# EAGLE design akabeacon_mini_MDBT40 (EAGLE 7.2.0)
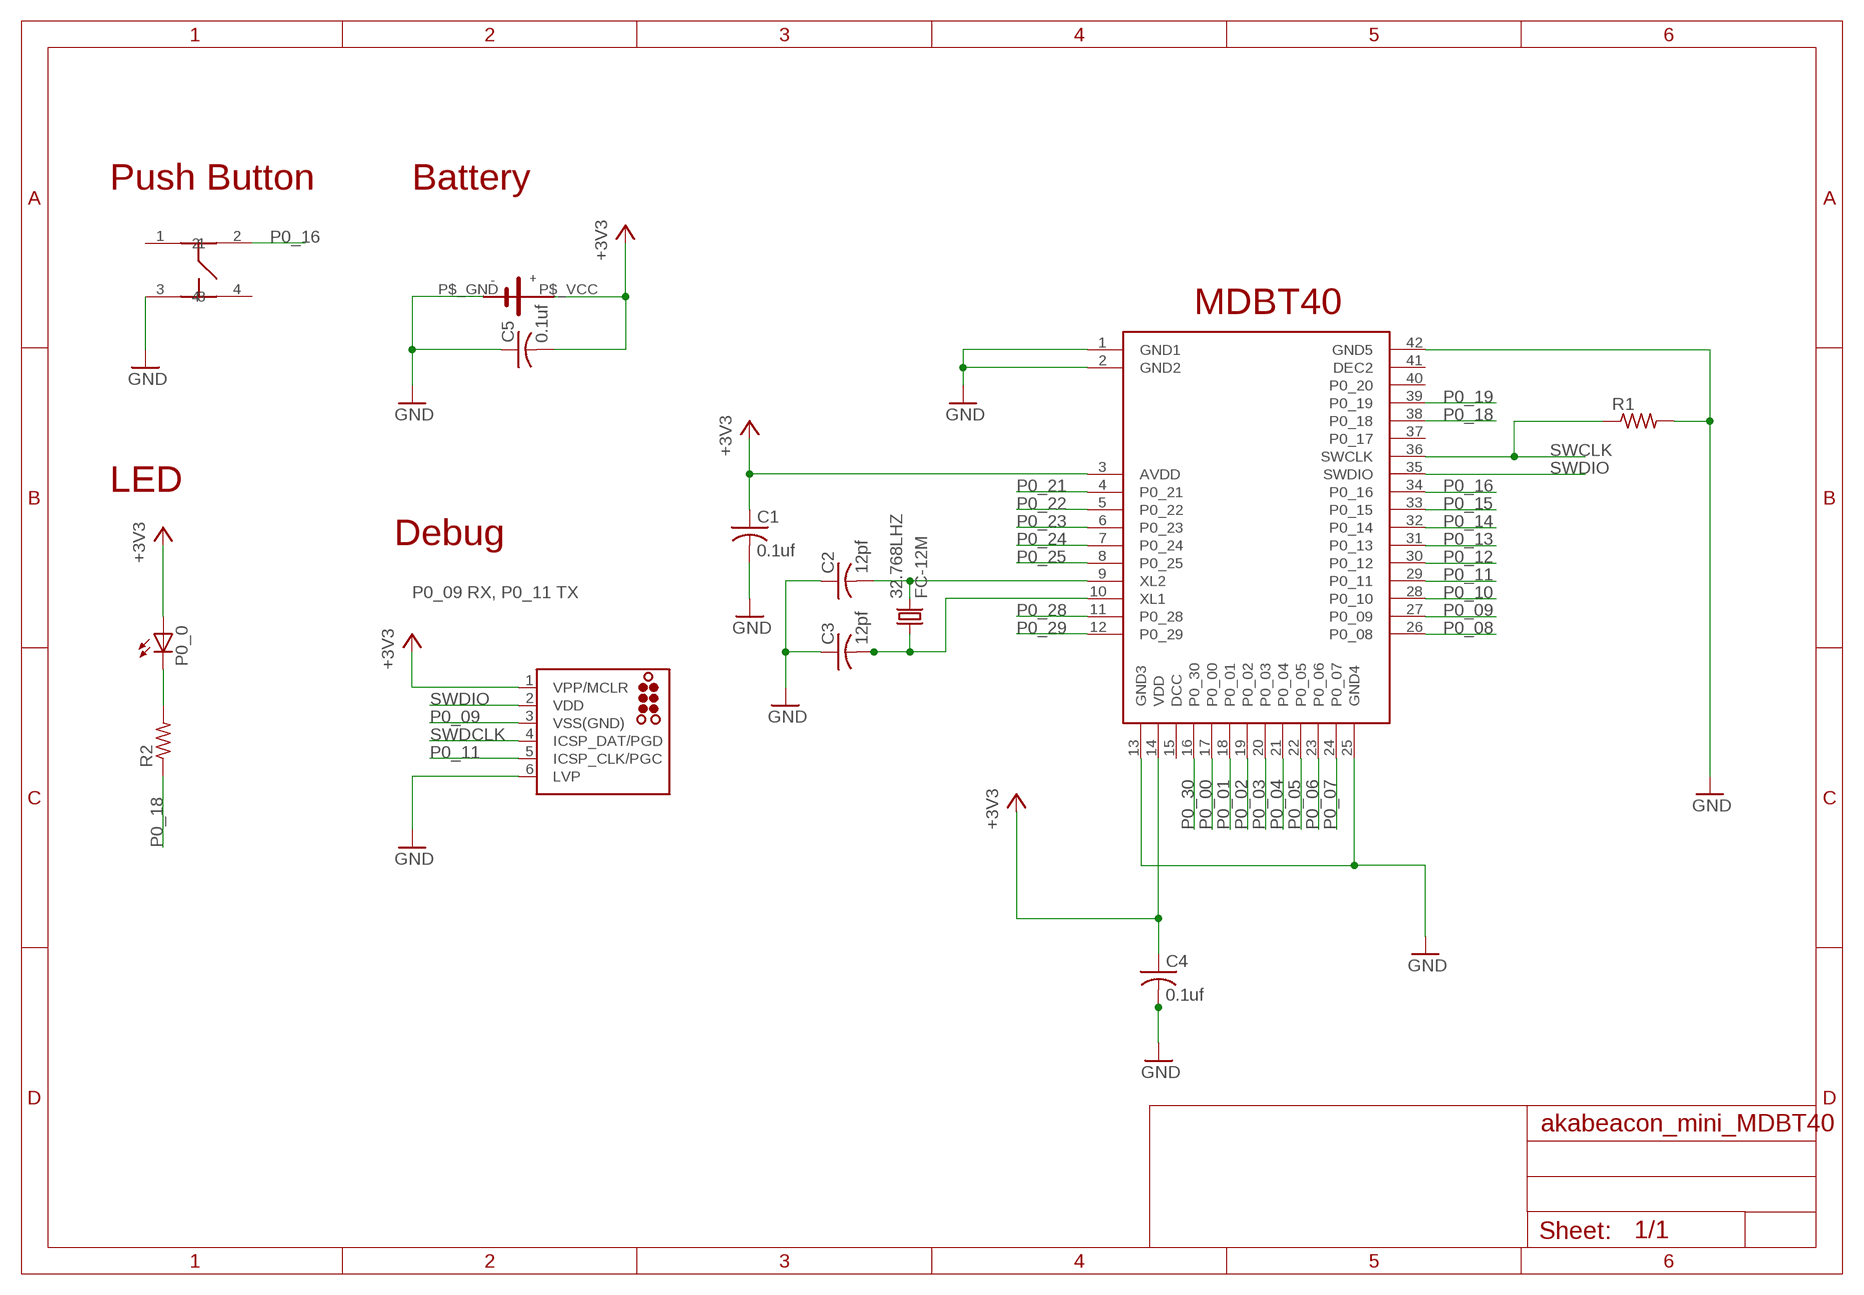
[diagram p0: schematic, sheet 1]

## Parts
32.768LHZ  FC-12M  [FC-12M]
C1  0.1uf  C-USC0603  [C0603]
C2  12pf  C-USC0603  [C0603]
C3  12pf  C-USC0603  [C0603]
C4  0.1uf  C-USC0603  [C0603]
C5  0.1uf  C-USC0603  [C0603]
J2  TC2030-MCP  [TC2030-MCP]
P0_0  LEDCHIP-LED0603  [CHIP-LED0603]
R1  R-US_R0603  [R0603]
R2  R-US_R0603  [R0603]
U$1  RAYTAC-MDBT40  [RAYTAC-MDBT40]
U$3  SMTU2450-BOTTOM-MINI  [SMTU2450-BOTTOM-MINI]
U$5  SWICTH-4P(KMR2)  [SWITCH-4P(KMR2)]

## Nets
+3V3: C1.1 C4.1 C5.2 J2.1(VPP/MCLR) P0_0.A U$1.3(AVDD) U$1.14(VDD) U$3.P$_VCC
GND: C1.2 C2.1 C3.1 C4.2 C5.1 J2.6(LVP) R1.2 U$1.1(GND1) U$1.2(GND2) U$1.13(GND3) U$1.25(GND4) U$1.42(GND5) U$3.P$_GND U$5.3
LED1: P0_0.C R2.2
N$7: 32.768LHZ.2 C2.2 U$1.9(XL2)
N$8: 32.768LHZ.1 C3.2 U$1.10(XL1)
P0_00: U$1.17(P0_00)
P0_01: U$1.18(P0_01)
P0_02: U$1.19(P0_02)
P0_03: U$1.20(P0_03)
P0_04: U$1.21(P0_04)
P0_05: U$1.22(P0_05)
P0_06: U$1.23(P0_06)
P0_07: U$1.24(P0_07)
P0_08: U$1.26(P0_08)
P0_09: J2.3(VSS(GND)) U$1.27(P0_09)
P0_10: U$1.28(P0_10)
P0_11: J2.5(ICSP_CLK/PGC) U$1.29(P0_11)
P0_12: U$1.30(P0_12)
P0_13: U$1.31(P0_13)
P0_14: U$1.32(P0_14)
P0_15: U$1.33(P0_15)
P0_16: U$1.34(P0_16) U$5.2
P0_18: R2.1 U$1.38(P0_18)
P0_19: U$1.39(P0_19)
P0_21: U$1.4(P0_21)
P0_22: U$1.5(P0_22)
P0_23: U$1.6(P0_23)
P0_24: U$1.7(P0_24)
P0_25: U$1.8(P0_25)
P0_28: U$1.11(P0_28)
P0_29: U$1.12(P0_29)
P0_30: U$1.16(P0_30)
SWCLK: R1.1 U$1.36(SWCLK)
SWDCLK: J2.4(ICSP_DAT/PGD)
SWDIO: J2.2(VDD) U$1.35(SWDIO)
Unconnected: U$1.15(DCC) U$1.37(P0_17) U$1.40(P0_20) U$1.41(DEC2) U$5.1 U$5.4

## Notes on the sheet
- Push Button | Battery
- MDBT40
- LED
- Debug
- P0_09 RX, P0_11 TX

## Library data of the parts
32.768LHZ = crystal:FC-12M: kHz RANGE CRYSTAL UNIT
C1-C5 = adafruit:C-US: CAPACITOR, American symbol
J2 = tag-connect:TC2030: TAG-CONNECT ICSP Connector Manufacturer: Tag-Connect Cable for easy In-Circuit Serial Programming. Designed for Microchip ICD2, suitable for many others. Two variants - one "with legs" (for hands-free fit on PCB) and another "without legs" for quick programming. PADDescription 1MCLR/Vpp 2Vdd 3GND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
P0_0 = led:LED: LED
R1 R2 = adafruit:R-US_: RESISTOR, American symbol
U$1 = gclueBT:RAYTAC-MDBT40
U$3 = gclue:SMTU2450-BOTTOM-MINI
U$5 = gclue-test:SWICTH-4P(KMR2)

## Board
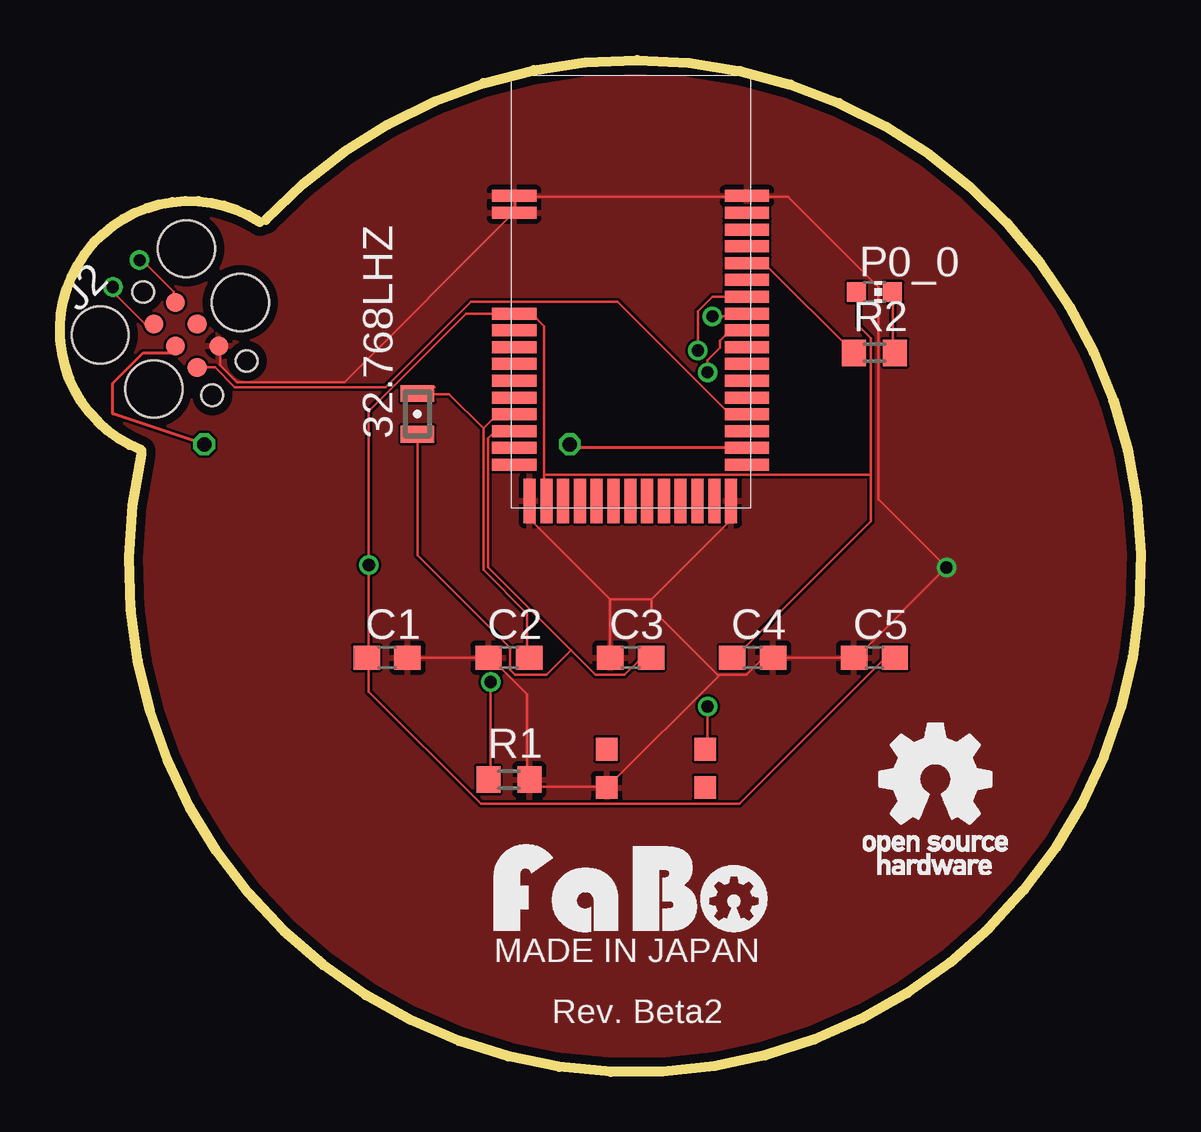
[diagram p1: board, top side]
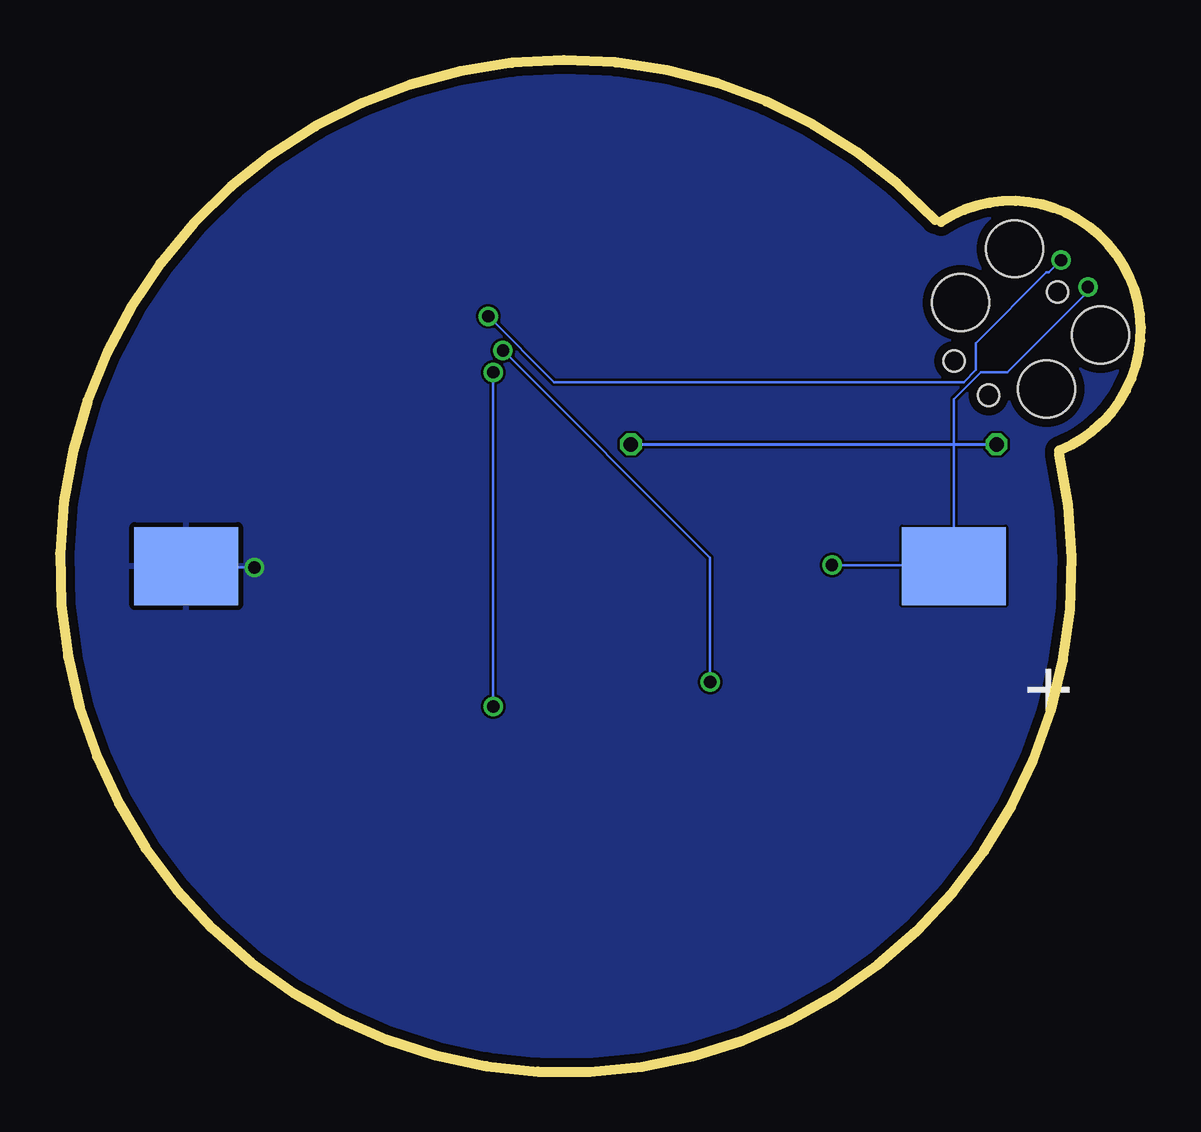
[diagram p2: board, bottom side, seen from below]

Size 45.05 x 42.16 mm. Coordinates in mm from the lower left corner, seen from the top.
Outline: 8.58,35.5 arc-330 3.4,25.74
Outline: 3.4,25.9 arc-191 8.32,35.42
Copper layers (1*16): Top 0.035mm / dielectric 1.5mm / Bottom 0.035mm
Design rules "default *": minimum track width 4mil, minimum drill 20mil, track to track 4mil, track to pad 4mil, pad to pad 4mil, via to via 4mil, smd to smd 4mil, copper to edge 15mil, drill to drill 5mil, minimum pad ring 8mil, minimum via ring 6mil, stop-mask expansion 4mil, vias tented up to drill 0mil, thermal gap 8mil

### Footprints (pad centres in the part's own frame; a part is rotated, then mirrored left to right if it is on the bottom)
FC-12M = smd 0.7 x 1.4: 1 -0.85,0; 2 0.85,0
C0603 = smd 1.1 x 1: 1 -0.85,0; 2 0.85,0
TC2030-MCP = smd 0.787 x 0.787: 1 1.27,-0.635; 2 1.27,0.635; 3 2.54,-0.635; 4 2.54,0.635; 5 3.81,-0.635; 6 3.81,0.635 | hole 0.889: 0,0; 5.08,-1.016; 5.08,1.016 | hole 2.375: 0,2.54; 0,-2.54; 3.175,-2.54; 3.175,2.54
CHIP-LED0603 = smd 0.8 x 0.8: A 0,-0.75; C 0,0.75
R0603 = smd 1 x 1.1: 1 -0.85,0; 2 0.85,0
RAYTAC-MDBT40 = smd 1.85 x 0.5: 1 -4.86,4; 2 -4.86,3.3; 3 -4.86,-0.9; 4 -4.86,-1.6; 5 -4.86,-2.3; 6 -4.86,-3; 7 -4.86,-3.7; 8 -4.86,-4.4; 9 -4.86,-5.1; 10 -4.86,-5.8; 11 -4.86,-6.5; 12 -4.86,-7.2; 26 4.84,-7.2; 27 4.84,-6.5; 28 4.84,-5.8; 29 4.84,-5.1; 30 4.84,-4.4; 31 4.84,-3.7; 32 4.84,-3; 33 4.84,-2.3; 34 4.84,-1.6; 35 4.84,-0.9; 36 4.84,-0.2; 37 4.84,0.5; 38 4.84,1.2; 39 4.84,1.9; 40 4.84,2.6; 41 4.84,3.3; 42 4.84,4 | smd 0.5 x 1.85: 13 -4.22,-8.71; 14 -3.52,-8.71; 15 -2.82,-8.71; 16 -2.12,-8.71; 17 -1.42,-8.71; 18 -0.72,-8.71; 19 -0.02,-8.71; 20 0.68,-8.71; 21 1.38,-8.71; 22 2.08,-8.71; 23 2.78,-8.71; 24 3.48,-8.71; 25 4.18,-8.71
SMTU2450-BOTTOM-MINI = smd 3.251 x 4.318 bottom: P$_GND 0,-16; P$_VCC 0,16
SWITCH-4P(KMR2) = smd 0.9 x 0.95: 1 -1,0; 2 3.1,0; 3 -1,-1.6; 4 3.1,-1.6

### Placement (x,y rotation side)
32.768LHZ  14.9,27.42 90 top
C1  13.63,17.26 0 top
C2  18.71,17.26 0 top
C3  23.79,17.26 0 top
C4  28.87,17.26 0 top
C5  33.95,17.26 0 top
J2  3.47,32.5 315 top
P0_0  33.95,32.5 270 top
R1  18.71,12.18 0 top
R2  33.95,29.96 0 top
U$1  23.79,32.5 0 top
U$2  [LOGO_FABO_M]  23.79,5.83 0 top
U$3  23.79,21.07 90 top
U$4  [LOGO_OSHW_T_M]  36.49,12.18 0 top
U$5  23.79,13.45 0 top

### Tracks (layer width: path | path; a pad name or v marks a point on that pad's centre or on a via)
+3V3  (via drill 0.51)
  Top 0.102: v2.2,32.7 2.2,32.5 3.52,31.18 3.83,31.18 J2.1 | 33.8,24.88 33.8,22.95 28.11,17.26 C4.1 | 33.8,24.88 33.8,30.57 33.29,31.08 33.29,32.5 P0_0.A | 12.87,17.26 v12.87,21.12 12.87,27.52 16.94,31.59 18.87,31.59 U$1.3 18.97,31.59 19.68,31.59 20.19,31.08 20.19,24.88 | C5.2 34.41,17.26 28.31,11.16 17.55,11.16 12.87,15.84 12.87,17.26 | 12.87,17.26 C1.1 | 20.19,24.88 20.19,23.86 U$1.14 | 20.19,24.88 33.8,24.88
  Bottom 0.102: v2.2,32.7 2.2,32.5 5.56,29.15 6.67,29.15 7.79,28.03 7.79,21.12 U$3.P$_VCC 7.89,21.12 v12.87,21.12
GND  (via drill 0.51)
  Top 0.102: J2.6 6.67,30.16 6.67,29.45 7.39,28.74 11.86,28.74 18.87,35.75 U$1.2 18.97,35.85 18.97,36.46 | 18.97,36.46 28.62,36.46 U$1.42 28.72,36.46 30.35,36.46 34.11,32.7 34.11,23.86 v36.95,21.02 33.19,17.26 C5.1 C4.2 29.33,17.26 28.62,16.55 27.5,16.55 | 18.97,36.46 U$1.1 | C1.2 C2.1 17.95,17.26 19.48,15.74 19.48,12.18 R1.2 19.58,12.18 19.88,11.88 22.73,11.88 U$5.3 22.83,11.88 27.5,16.55 | 22.93,19.7 22.93,17.26 C3.1 | 22.93,19.7 19.58,23.05 19.58,23.76 U$1.13 | 24.66,19.7 27.91,22.95 27.91,23.76 U$1.25 | 22.93,19.7 24.66,19.7 | 27.5,16.55 27.4,16.55 24.66,19.29 24.66,19.7
  Bottom 0.102: v36.95,21.02 39.69,21.02 U$3.P$_GND
  pour Bottom: -0.34,-0.52 46.65,-0.52 46.65,42.66 -0.34,42.66
  pour Top: -0.34,-0.52 46.65,-0.52 46.65,42.66 -0.34,42.66
LED1
  Top 0.102: P0_0.C 34.72,32.5 34.72,29.96 R2.2
N$1
  Top 0.102: 15.61,28.54 15.61,28.53
N$7
  Top 0.102: 17.65,26.81 17.65,20.92 19.48,19.09 19.48,17.26 C2.2 | 17.65,26.81 18.15,27.32 18.87,27.32 U$1.9 | 17.65,26.81 16.22,28.23 14.9,28.23 32.768LHZ.2
N$8
  Top 0.102: C3.2 24.25,17.26 23.54,16.55 22.32,16.55 21.3,17.57 | 21.3,17.57 17.85,21.02 17.85,26.4 18.05,26.61 18.87,26.61 U$1.10 | 32.768LHZ.1 14.9,21.53 18.76,17.67 18.76,16.75 18.97,16.55 20.29,16.55 21.3,17.57
P0_09  (via drill 0.6)
  Top 0.127: U$1.27 21.25,26 v21.25,26.15 | v6.01,26.15 2.2,27.42 2.2,28.69 3.47,29.96 4.74,29.96 J2.3
  Bottom 0.127: v21.25,26.15 v6.01,26.15
P0_11
  Top 0.102: J2.5 5.76,29.35 6.47,29.35 7.28,28.54 13.58,28.54 17.14,32.09 23.23,32.09 27.91,27.42 28.62,27.42 U$1.29
P0_16  (via drill 0.51)
  Top 0.102: v26.99,15.23 26.99,13.5 U$5.2 | v26.99,29.15 26.99,29.66 27.5,30.16 27.5,30.47 27.91,30.87 28.62,30.87 U$1.34
  Bottom 0.102: v26.99,29.15 v26.99,15.23
P0_18
  Top 0.102: R2.1 33.09,29.96 29.43,33.62 28.72,33.62 U$1.38
SWCLK  (via drill 0.51)
  Top 0.102: v17.95,16.24 17.95,12.18 R1.1 | v26.59,30.06 26.59,31.69 27.2,32.3 28.62,32.3 U$1.36
  Bottom 0.102: v17.95,16.24 17.95,21.43 v26.59,30.06
SWDIO  (via drill 0.51)
  Top 0.102: v3.32,33.82 3.42,33.82 4.74,32.5 4.74,32.09 J2.2 | v27.2,31.48 28.52,31.48 28.62,31.59 U$1.35
  Bottom 0.102: v3.32,33.82 3.83,33.31 3.93,33.31 6.88,30.37 6.88,29.25 7.39,28.74 24.45,28.74 v27.2,31.48

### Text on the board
tPlace: MADE IN JAPAN | Rev. Beta2

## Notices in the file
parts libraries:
SparkFun: Licensing: CC v3.0 Share-Alike You are welcome to use this library for commercial purposes.
tag-connect: ©2009 ROFA.cz - modified and updated by Robert Darlington ‹rdarlington@gmail.com›
